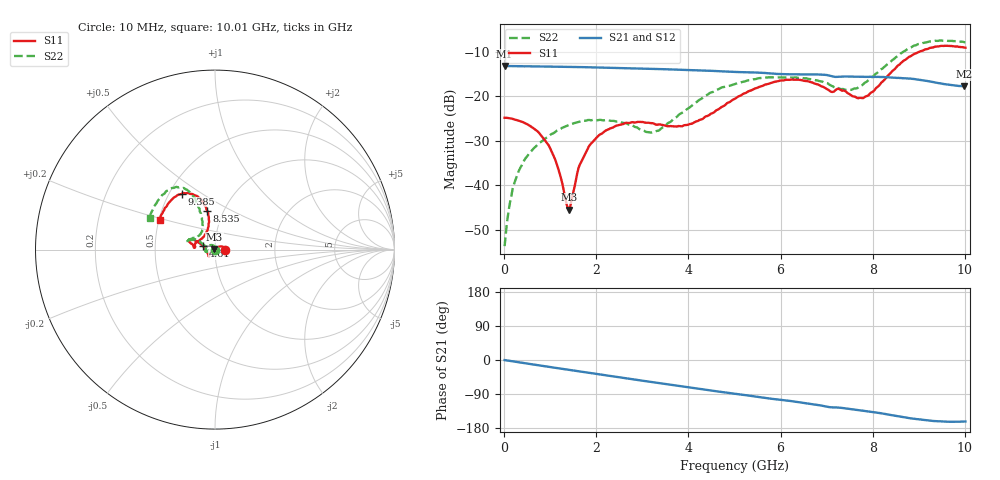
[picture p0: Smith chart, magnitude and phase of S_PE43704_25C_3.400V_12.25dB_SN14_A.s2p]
! Device ID: PE43704
! Dir: z:\PE43704\PE43704_Char_1_20130516\PE43704\AMB\3p400V\12p25dB
! Serial: 14
! Insertion: A
! Impedance: 50 ohm
! Temp: Amb
! VDD: 3.400V
! Attenuation Step: 12.25dB
! IDD: 1.140243e-01mA
#  Hz  S  RI  R  50
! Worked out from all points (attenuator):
!   401 points, 10 MHz to 10.01 GHz, reference 50 ohm
!   highest |S21| = -13.21 dB at 10 MHz (marker M1); lowest = -17.8 dB at 9.985 GHz (marker M2)
!   lowest |S11| = -45.5 dB at 1.41 GHz (marker M3), VSWR 1.01, Z = 49.6 + j0.353 ohm
!   |S11| at or under -10 dB: start of sweep to 9.008 GHz
!   |S22| runs from -53.7 to -7.5 dB; largest |S21 - S12| = 0.0016
!   S11 on the Smith chart (normalised r, x): 10 MHz: 1.12, +0.00; 4.61 GHz: 0.87, +0.03; 8.535 GHz: 0.84, +0.38; 9.385 GHz: 0.58, +0.42; 10.01 GHz: 0.50, +0.19
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1e7  0.0572 0.00017  0.2186 -0.000824  0.2186 -0.000767  0.00202 0.000405
1.85e8  0.0552 0.0059  0.2175 -0.0135  0.2175 -0.0135  0.00153 0.00904
4.1e8  0.0494 0.0124  0.2148 -0.0299  0.215 -0.0292  -0.00268 0.0176
9.85e8  0.0212 0.0166  0.2045 -0.0675  0.2045 -0.0674  -0.0258 0.0253
1.16e9  0.0105 0.0123  0.1999 -0.0787  0.1999 -0.0786  -0.0348 0.0221
1.41e9  -0.00393 0.00356  0.192 -0.0938  0.192 -0.0937  -0.0452 0.015
1.685e9  -0.0171 -0.0077  0.1822 -0.1095  0.1822 -0.1094  -0.0526 0.00482
1.885e9  -0.0244 -0.0161  0.174 -0.1201  0.1741 -0.12  -0.0536 -0.00245
2.26e9  -0.0306 -0.0292  0.1572 -0.1384  0.1572 -0.1383  -0.0524 -0.0107
3.36e9  -0.036 -0.0321  0.0984 -0.1765  0.0986 -0.1764  -0.0408 0.00604
4.01e9  -0.0476 -0.00744  0.0601 -0.1873  0.0604 -0.1874  -0.0674 0.03
4.61e9  -0.0671 0.0191  0.0247 -0.1901  0.0251 -0.19  -0.104 0.055
5.01e9  -0.0865 0.0364  0.00324 -0.1875  0.00329 -0.1875  -0.1262 0.0538
5.96e9  -0.1365 0.058  -0.0446 -0.1724  -0.044 -0.1727  -0.1543 0.0513
6.685e9  -0.138 0.0377  -0.0777 -0.1576  -0.078 -0.1577  -0.1454 0.0524
7.36e9  -0.1108 0.0333  -0.0999 -0.133  -0.0997 -0.1328  -0.0942 0.075
7.735e9  -0.0672 0.0682  -0.1128 -0.1212  -0.1125 -0.1214  -0.0717 0.1093
8.36e9  -0.0345 0.1729  -0.1324 -0.0946  -0.1319 -0.0951  -0.0855 0.2222
8.535e9  -0.0431 0.2143  -0.1365 -0.0845  -0.1359 -0.0856  -0.1037 0.2641
9.385e9  -0.1847 0.3114  -0.1345 -0.045  -0.1348 -0.0447  -0.2522 0.335
9.985e9  -0.3042 0.1777  -0.1234 -0.0392  -0.1239 -0.0392  -0.3598 0.1859
1.001e10  -0.3089 0.1674  -0.1236 -0.0397  -0.1244 -0.0399  -0.3636 0.1776
